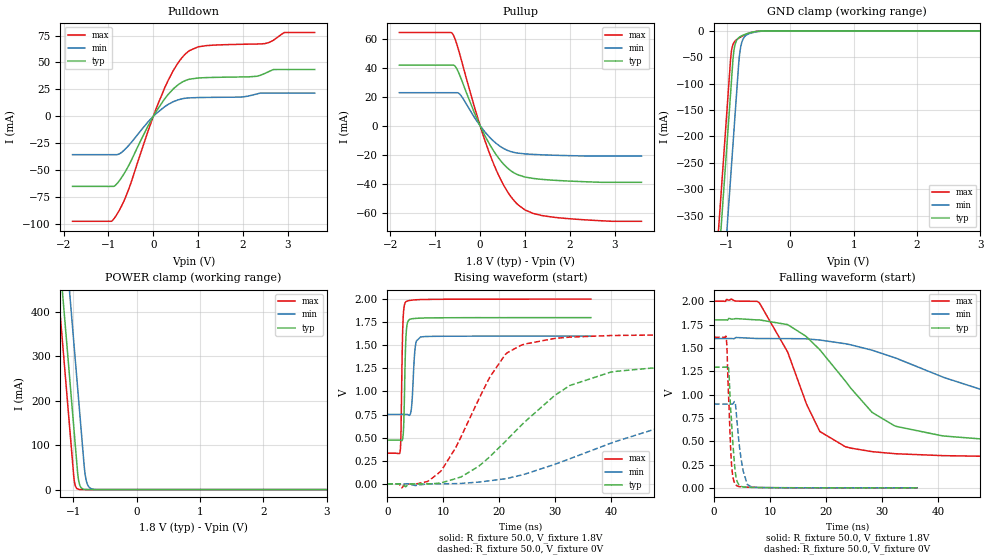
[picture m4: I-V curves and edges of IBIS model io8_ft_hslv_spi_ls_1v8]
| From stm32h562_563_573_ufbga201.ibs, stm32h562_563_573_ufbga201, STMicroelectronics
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[Model]   io8_ft_hslv_spi_ls_1v8
Model_type I/O
Polarity   Non-Inverting
Enable   Active-Low
| CAP_THRESHOLD on pad IOFT is "UDTCAPC" :
| Rising=20.0% of vddiom   Falling=80.0% of vddiom
| C_comp min and max val. don't necessarily correlate with the min and max pvt
| but are the smallest and greatest pad capacitance found.
| var   typ   min   max
C_comp   4.56162pF  4.45450pF  4.74984pF
|C_comp_pullup   2.85880pF  2.67905pF  2.77985pF
|C_comp_pulldown   1.70282pF  1.77545pF  1.96999pF
Vinl = 480.0mV
Vinh = 1.4V
Vmeas = 900.0mV   | Reference voltage for timing measurements
Cref  = 50.0pF   | Timing specification test load capacitance value
Rref  = 100.0MOhm   | Timing specification test load resistance value
Vref  = 900.0mV   | Timing specification test load voltage
[Model Spec]
| TIME_THRESHOLD on pin ZIV11 is "CMOS" :
| Rising=40.0% of vdd   Falling=60.0% of vdd
Vinl 703.80000mV 631.80000mV 784.80000mV
Vinh 1.06220V 937.20000mV 1.16620V
| variable   typ   min   max
[Temperature Range] 25.0 125.0 -40.0
| variable   typ   min   max
[Voltage Range] 1.8V 1.6V 2.0V
| variable   typ   min   max
[POWER Clamp Reference] 1.8V 1.6V 2.0V
| variable   typ   min   max
[GND Clamp Reference] 0V 0V 0V
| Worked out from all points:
|   slope of the pulldown table from 0 to 0.27 V, typ, clamps not added: 15.8 ohm
|   slope of the pullup table from 0 to 0.27 V, typ, clamps not added: 17.1 ohm
|   GND clamp passes 1 mA (typ) near -0.52 V on its own axis
|   POWER clamp passes 1 mA (typ) near -0.84 V on its own axis
|   rising waveform, R_fixture 50.0, V_fixture 1.8V: 20-80 % time 308ps typ, 458ps min, 279ps max; typ from 0.474 V to 1.8 V
|   falling waveform, R_fixture 50.0, V_fixture 1.8V: 20-80 % time 12.2ns typ, 28.6ns min, 7.27ns max; typ from 1.8 V to 0.474 V
|   rising waveform, R_fixture 50.0, V_fixture 0V: 20-80 % time 14.2ns typ, 28.3ns min, 8.33ns max; typ from 0 V to 1.29 V
|   falling waveform, R_fixture 50.0, V_fixture 0V: 20-80 % time 836ps typ, 1.11ns min, 632ps max; typ from 1.29 V to 0 V
[POWER Clamp]
-1.8V     1.518A     1.709A     1.407A
-1.23V    548.8mA    740.2mA    437.5mA
-1.16V    429.8mA    621.2mA    318.5mA
-1.05V    242.8mA    434.2mA    131.5mA
-980mV    123.8mA    315.2mA    17.95mA
-930mV    38.81mA    230.2mA    1.49mA
-910mV    17.82mA    196.2mA    550.8uA
-890mV    8.18mA     162.2mA    203.5uA
-810mV    363.5uA    33.6mA     3.797uA
-770mV    76.62uA    10.47mA    518.8nA
-710mV    7.417uA    1.822mA    26.38nA
3.6V      0A         0A         0A
[GND Clamp]
-1.8V     -1.581A    -1.742A    -1.516A
-1.24V    -628.8mA   -789.9mA   -564.1mA
-1.05V    -305.8mA   -466.9mA   -241.1mA
-940mV    -118.8mA   -279.9mA   -54.1mA
-930mV    -101.8mA   -262.9mA   -41.86mA
-900mV    -51.51mA   -211.9mA   -25.34mA
-880mV    -32.22mA   -177.9mA   -21mA
-810mV    -13.02mA   -59.5mA    -13.82mA
-770mV    -9.8mA     -24.99mA   -11mA
-680mV    -5.275mA   -7.288mA   -5.917mA
-400mV    -107uA     -349.1uA   -42.51uA
3.6V      5.392nA    968.2nA    261.3pA
| variable   typ   min   max
[Pullup Reference] 1.8V 1.6V 2.0V
| variable   typ   min   max
[Pulldown Reference] 0V 0V 0V
[Pullup]
-1.8V     41.69mA    22.72mA    64.13mA
-610mV    41.69mA    22.72mA    63.15mA
-540mV    40.22mA    22.72mA    58.1mA
-440mV    33.7mA     21.26mA    47.77mA
-120mV    8.364mA    5.385mA    12.19mA
70mV      -4.507mA   -2.839mA   -6.693mA
240mV     -14.24mA   -8.79mA    -21.45mA
540mV     -26.97mA   -15.93mA   -41.71mA
850mV     -33.87mA   -18.89mA   -54.53mA
1.18V     -36.29mA   -19.75mA   -60.37mA
1.56V     -37.38mA   -20.24mA   -62.7mA
3.6V      -38.97mA   -20.89mA   -65.81mA
[Pulldown]
-1.8V     -65.02mA   -35.56mA   -97.42mA
-940mV    -65.02mA   -35.56mA   -97.42mA
-850mV    -64.17mA   -35.56mA   -93.5mA
-570mV    -47.32mA   -28.01mA   -70.04mA
-120mV    -9.088mA   -5.279mA   -14.07mA
250mV     16.04mA    8.832mA    26.05mA
550mV     29.17mA    15.25mA    49.41mA
780mV     34.17mA    17.07mA    60.14mA
1.18V     35.97mA    17.56mA    65.65mA
2.49V     39.87mA    21.59mA    67.54mA
2.92V     43.47mA    21.59mA    77.77mA
3.6V      43.47mA    21.59mA    77.77mA
[Ramp]
dV/dt_r 775.80952mV/14.09313ns 538.8744mV/28.15219ns 968.324mV/8.00078ns
dV/dt_f 795.78715mV/11.7312ns 508.95919mV/28.16477ns 1.00099V/6.50855ns
R_load = 50.0
| Removed startup time: 0s 0s 0s  .
| Removed end time: 36.4ns.
[Rising Waveform]
R_fixture   = 50.0
V_fixture   = 1.8V
V_fixture_min = 1.6V
V_fixture_max = 2.0V
0s        473.7mV    751.7mV    331.7mV
2.3ns     473.8mV    751.7mV    348.5mV
2.45ns    471.1mV    751.7mV    549.9mV
2.8ns     506.4mV    751.8mV    1.741V
2.95ns    652.8mV    751.8mV    1.889V
3.35ns    1.601V     752mV      1.972V
4.2ns     1.785V     770.4mV    1.987V
5ns       1.791V     1.48V      1.992V
5.95ns    1.794V     1.591V     1.995V
36.4ns    1.8V       1.6V       2V
| Removed startup time: 0s 0s 0s  .
| Removed end time: 399.4ns.
[Falling Waveform]
R_fixture   = 50.0
V_fixture   = 1.8V
V_fixture_min = 1.6V
V_fixture_max = 2.0V
0s        1.8V       1.6V       2V
8.15ns    1.8V       1.6V       1.978V
13.15ns   1.749V     1.6V       1.456V
16.55ns   1.617V     1.597V     893.2mV
18.9ns    1.48V      1.584V     604.2mV
28.25ns   808.3mV    1.475V     388mV
32.2ns    667mV      1.397V     366.8mV
53.95ns   505.1mV    966.7mV    335.5mV
89.65ns   477mV      795.7mV    331.8mV
399.4ns   473.7mV    751.7mV    331.7mV
| Removed startup time: 0s 0s 0s  .
| Removed end time: 399.3ns.
[Rising Waveform]
R_fixture   = 50.0
V_fixture   = 0V
V_fixture_min = 0V
V_fixture_max = 0V
0s        134.7nV    547.1nV    93.87nV
2.6ns     -3.265mV   -4.372uV   -43.57mV
9.6ns     10.47mV    82.7uV     139.6mV
16.3ns    188.1mV    18.69mV    909.9mV
21.5ns    483.6mV    59.9mV     1.421V
32.6ns    1.064V     271.3mV    1.588V
40.8ns    1.218V     458.3mV    1.607V
57.1ns    1.28V      723.6mV    1.613V
89.7ns    1.292V     876.6mV    1.614V
399.3ns   1.293V     898.1mV    1.614V
| Removed startup time: 0s 0s 0s  .
| Removed end time: 36.4ns.
[Falling Waveform]
R_fixture   = 50.0
V_fixture   = 0V
V_fixture_min = 0V
V_fixture_max = 0V
0s        1.293V     898.2mV    1.614V
2.15ns    1.293V     898.2mV    1.622V
2.3ns     1.296V     898.3mV    1.497V
2.6ns     1.277V     898.3mV    970.5mV
3.1ns     730.5mV    898.1mV    269.3mV
3.7ns     223.7mV    924.2mV    48.33mV
4ns       94.6mV     781.2mV    25.68mV
5.2ns     10.28mV    180mV      9.466mV
6.7ns     5.251mV    9.962mV    5.754mV
36.4ns    126.2uV    249.7uV    65.84uV
